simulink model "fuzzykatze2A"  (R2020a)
settings: Solver=ode45  StartTime=0.0  StopTime=100  RelTol=1e-5  EnableMultiTasking=on
libraries: libregler2 x7

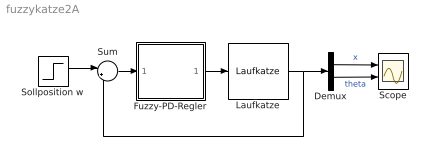
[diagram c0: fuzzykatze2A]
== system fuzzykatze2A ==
  Demux : Demux  Outputs=2
  Fuzzy-PD-Regler : Subsystem  mask{bx=1, bth=0.001, bv=0.01, hmax=10, Kp=60}
      mask prompts: bx "Breite Position"; bth "Breite Seilwinkel"; bv "Breite Geschwindigkeit"; hmax "Stabilisierungsfaktor"; Kp "Regelverstaerkung"
  Laufkatze : libregler2/Laufkatze  mk=100  ml=500  l=3  g=9.81
  Scope : Scope  NumInputPorts=2
  Sollposition w : Step  Time=5  Before=[0,0]  After=[10,0]  SampleTime=0
  Sum : Sum  Inputs=|+-  SaturateOnIntegerOverflow=on
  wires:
  Fuzzy-PD-Regler/1(u) -> Laufkatze/1
  Demux/1 -> Scope/1  "x"
  Demux/2 -> Scope/2  "theta"
  Laufkatze/1 -> Demux/1, Sum/2
  Sollposition w/1 -> Sum/1
  Sum/1 -> Fuzzy-PD-Regler/1(e)

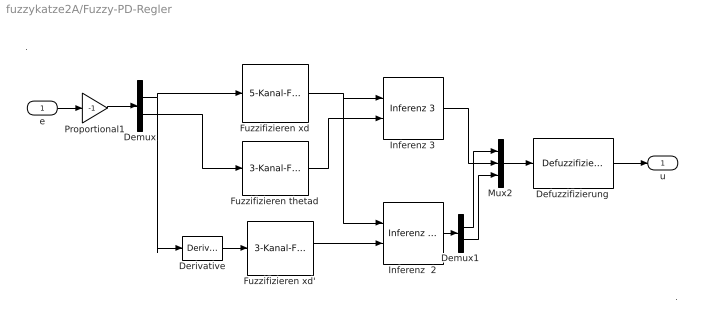
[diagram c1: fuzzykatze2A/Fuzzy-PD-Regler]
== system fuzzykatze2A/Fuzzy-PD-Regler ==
  note: .
  note: .
  e : Inport
  Defuzzifizierung : libregler2/Defuzzifizierung  h=[-hmax, -1, 0, 1, hmax]*Kp
  Demux : Demux  Outputs=2
  Demux1 : Demux  Outputs=2
  Derivative : Derivative
  Fuzzifizieren thetad : libregler2/3-Kanal-Fuzzifizierer  w=bth  offset=0
  Fuzzifizieren xd : libregler2/5-Kanal-Fuzzifizierer  w=bx  offset=0
  Fuzzifizieren xd' : libregler2/3-Kanal-Fuzzifizierer  w=bv  offset=0
  Inferenz  2 : libregler2/Inferenz  2  M=[2 0 0; 2 0 0; 0 0 0; 0 0 1; 0 0 1]
  Inferenz 3 : libregler2/Inferenz 3  M=[3 3 3; 2 3 3; 1 2 3; 1 1 2; 1 1 1]
  Mux2 : Mux  Inputs=3
  Proportional1 : Gain  Gain=-1  SaturateOnIntegerOverflow=on
  u : Outport
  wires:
  Fuzzifizieren xd/1 -> Inferenz  2/1, Inferenz 3/1
  Demux/1 -> Fuzzifizieren xd/1, Derivative/1
  Demux/2 -> Fuzzifizieren thetad/1
  e/1 -> Proportional1/1
  Derivative/1 -> Fuzzifizieren xd'/1
  Inferenz 3/1 -> Mux2/2
  Defuzzifizierung/1 -> u/1
  Mux2/1 -> Defuzzifizierung/1
  Proportional1/1 -> Demux/1
  Inferenz  2/1 -> Demux1/1
  Demux1/1 -> Mux2/1
  Demux1/2 -> Mux2/3
  Fuzzifizieren xd'/1 -> Inferenz  2/2
  Fuzzifizieren thetad/1 -> Inferenz 3/2
